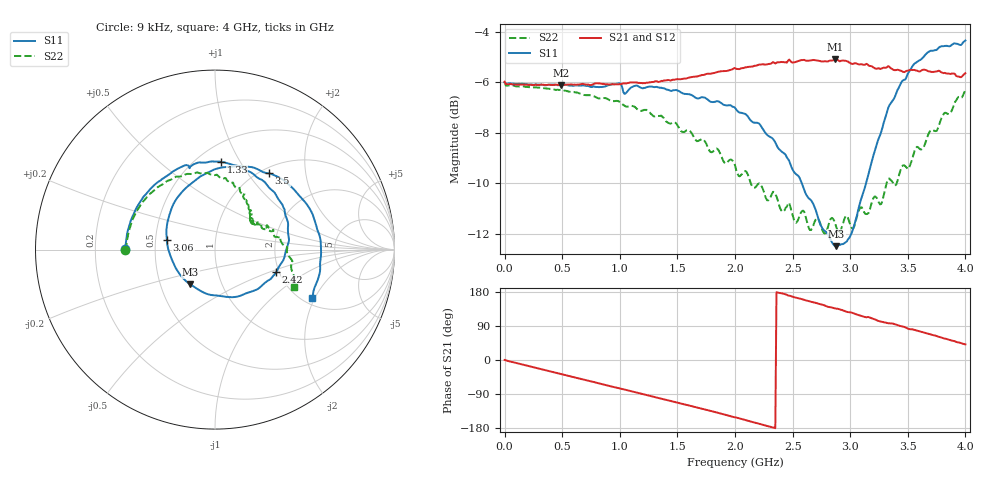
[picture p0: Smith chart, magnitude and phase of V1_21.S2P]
! ZVRE, 3.40
! symbol freq-unit parameter-type data-format keyword impedance-ohm
#  HZ  S  RI  R  50
! freq  reS11  imS11  reS21  imS21  reS12  imS12  reS22  imS22
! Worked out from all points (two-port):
!   401 points, 9 kHz to 4 GHz, reference 50 ohm
!   highest |S21| = -5.09 dB at 2.87 GHz (marker M1); lowest = -6.1 dB at 490 MHz (marker M2)
!   |S21| within 3 dB of the highest: start of sweep to end of sweep
!   lowest |S11| = -12.5 dB at 2.88 GHz (marker M3), VSWR 1.62, Z = 35.4 - j14.5 ohm
!   |S11| at or under -10 dB: 2.58 GHz to 3.138 GHz (557.8 MHz wide, 19.5 % of centre)
!   |S22| runs from -12.0 to -6.0 dB; largest |S21 - S12| = 0.023
!   S11 on the Smith chart (normalised r, x): 9 kHz: 0.33, +0.00; 1.33 GHz: 0.65, +0.83; 2.42 GHz: 1.93, -0.55; 3.06 GHz: 0.57, +0.07; 3.5 GHz: 1.09, +1.27; 4 GHz: 2.23, -1.91
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9000  -0.5004 0.0013  0.5024 0.000811  0.5027 -0.00202  -0.5009 -0.000186
4.900079e8  -0.4113 0.2743  0.3942 -0.2981  0.4001 -0.2967  -0.413 0.2513
6.700075e8  -0.344 0.354  0.3159 -0.3838  0.3218 -0.3823  -0.3502 0.3202
9.900068e8  -0.1772 0.4661  0.1334 -0.4782  0.1374 -0.4801  -0.2151 0.4059
1.330006e9  0.0321 0.4886  -0.0861 -0.4947  -0.0829 -0.4986  -0.0501 0.4267
1.340006e9  0.0385 0.4876  -0.0912 -0.4935  -0.0894 -0.4977  -0.048 0.427
1.720005e9  0.2665 0.3847  -0.3256 -0.4027  -0.3245 -0.4066  0.0994 0.3736
2.000004e9  0.3881 0.2199  -0.4684 -0.2575  -0.4672 -0.2613  0.1594 0.3039
2.210004e9  0.412 0.0491  -0.5316 -0.1106  -0.5319 -0.1159  0.197 0.2473
2.420004e9  0.3416 -0.1238  -0.5473 0.048  -0.5498 0.0472  0.1972 0.1963
2.670003e9  0.1268 -0.2612  -0.4938 0.2512  -0.5023 0.2444  0.203 0.1589
2.870003e9  -0.1253 -0.2017  -0.4004 0.3863  -0.4096 0.3787  0.2083 0.1607
2.880003e9  -0.1376 -0.1935  -0.3967 0.3899  -0.4037 0.3867  0.2051 0.1575
3.060002e9  -0.2682 0.0559  -0.2703 0.4732  -0.2725 0.4791  0.2346 0.1388
3.180002e9  -0.2309 0.2552  -0.1928 0.5037  -0.1978 0.5092  0.2497 0.1391
3.340001e9  0.0101 0.451  -0.0645 0.5337  -0.0656 0.5392  0.2963 0.129
3.430001e9  0.1713 0.4625  -0.000686 0.5287  -0.004 0.5401  0.3161 0.1016
3.500001e9  0.3014 0.4251  0.0643 0.5242  0.0537 0.5363  0.3268 0.0848
3.640001e9  0.4904 0.2771  0.1588 0.5064  0.1595 0.5144  0.3718 0.0372
3.750001e9  0.5692 0.1131  0.2376 0.4697  0.2401 0.4762  0.401 -0.0154
3.89e9  0.5859 -0.1088  0.33 0.4035  0.3401 0.4055  0.4289 -0.1191
4e9  0.5421 -0.2711  0.3934 0.3433  0.3991 0.3379  0.4377 -0.2078
